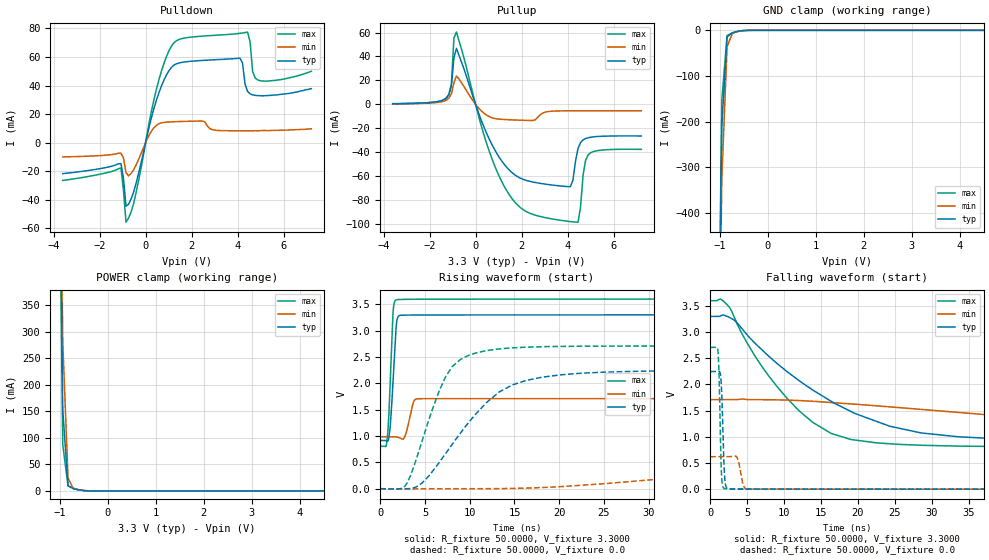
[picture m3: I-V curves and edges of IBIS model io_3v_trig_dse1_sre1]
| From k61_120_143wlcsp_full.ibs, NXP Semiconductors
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[Model]  io_3v_trig_dse1_sre1
|   Model io_3v_trig_dse1_sre1
| Library cells for typ/min/max conditions are connected as defined below:
|  pad - External Pad
|  ipp_do_3v - Core Input
|  ipp_obe_3v - Output Buffer Enable
|  esd_boost - vdd_s_3v
|  esd_trigger - vss_s_3v
|  ipp_ame_3v - vss_s_3v
|  ipp_dse_3v - vdd_s_3v
|  ipp_ina_3v - NC
|  ipp_ina_mux_3v - NC
|  ipp_ind_3v - NC
|  ipp_pue_3v - vss_s_3v
|  ipp_sre_3v - vdd_s_3v
|  tie_3v - vdd_s_3v
|  tie_hi - vdd_s_lv
|  vbuf_3v - vdd_s_3v
|  vdd_s_3v - vdd_s_3v
|  vdd_s_lv - vdd_s_lv
|  vss_bulk - vss_s_3v
|  vss_s_3v - vss_s_3v
| All other pins connected to ground
Model_type I/O
Polarity   Non-Inverting
Enable   Active-High
Vinl =   1.1550V
Vinh =   2.3100V
Vmeas =  1.6500V
Cref =   25.0000pF
Rref =   50.0000
Vref =   0.0V
C_comp   1.9033pF   1.7921pF   2.1182pF
[Temperature Range]   25.0000   0.1250k   -40.0000
[Voltage Range]   3.3000V   1.7100V   3.6000V
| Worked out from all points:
|   slope of the pulldown table from 0 to 0.495 V, typ, clamps not added: 16 ohm
|   slope of the pullup table from 0 to 0.495 V, typ, clamps not added: 19.9 ohm
|   GND clamp passes 1 mA (typ) near -0.54 V on its own axis
|   POWER clamp passes 1 mA (typ) near -0.53 V on its own axis
|   rising waveform, R_fixture 50.0000, V_fixture 3.3000: 20-80 % time 477ps typ, 573ps min, 395ps max; typ from 0.916 V to 3.3 V
|   rising waveform, R_fixture 50.0000, V_fixture 0.0: 20-80 % time 6.64ns typ, 30.7ns min, 3.47ns max; typ from 0 V to 2.25 V
|   falling waveform, R_fixture 50.0000, V_fixture 3.3000: 20-80 % time 14.8ns typ, 48ns min, 9.11ns max; typ from 3.3 V to 0.916 V
|   falling waveform, R_fixture 50.0000, V_fixture 0.0: 20-80 % time 304ps typ, 500ps min, 253ps max; typ from 2.25 V to 0 V
[Pulldown]
|Voltage   I(typ)   I(min)   I(max)
-3.6V     -21.69mA   -9.96mA    -26.46mA
-1.07V    -14.69mA   -7.404mA   -17.65mA
-850mV    -44.53mA   -20.93mA   -55.69mA
-520mV    -34.62mA   -18.99mA   -42.62mA
580mV     34.99mA    13.27mA    44.1mA
1.46V     55.81mA    14.78mA    72.31mA
4.1V      59.15mA    8.3mA      76.57mA
4.43V     35.88mA    8.3mA      77.43mA
4.54V     34.19mA    8.3mA      70.65mA
4.65V     33.46mA    8.3mA      49.92mA
4.87V     32.94mA    8.3mA      43.91mA
7.2V      37.8mA     9.7mA      50mA
[Pullup]
|Voltage   I(typ)   I(min)   I(max)
-3.6V     600uA      400uA      600uA
-1.27V    5.28mA     3.56mA     5.35mA
-1.05V    15.3mA     8.87mA     17.35mA
-940mV    39.22mA    18.09mA    55.5mA
-830mV    46.74mA    23.72mA    60.38mA
1.15V     -47.61mA   -12.48mA   -64.99mA
3.24V     -67.13mA   -5.816mA   -95.35mA
4.12V     -68.69mA   -5.32mA    -97.87mA
4.45V     -36.82mA   -5.29mA    -98.37mA
4.78V     -28.52mA   -5.28mA    -46.64mA
5V        -27.41mA   -5.28mA    -40.35mA
7.2V      -26.38mA   -5.36mA    -37.57mA
[GND_clamp]
|Voltage   I(typ)   I(min)   I(max)
-3.6V     -47.82A    -47.1A     -48.34A
-1.07V    -1.102A    -1.183A    -1.105A
-960mV    -210.7mA   -326mA     -154mA
-850mV    -14.47mA   -36.11mA   -11.11mA
-740mV    -5.262mA   -6.033mA   -5.843mA
-520mV    -636.9uA   -915.4uA   -467.5uA
-300mV    -2.578uA   -18.09uA   -370.9nA
7.2V      0A         0A         0A
[POWER_clamp]
|Voltage   I(typ)   I(min)   I(max)
-3.6V     36.98A     36.74A     37.19A
-1.05V    1.02A      1.161A     949.9mA
-940mV    152.3mA    280.6mA    87.35mA
-830mV    9.987mA    24.48mA    9.181mA
-720mV    4.227mA    4.408mA    5.116mA
-500mV    628.6uA    743.9uA    622.6uA
-390mV    66.57uA    164uA      29.9uA
7.2V      0A         0A         0A
[Ramp]
| variable   typ   min   max
dV/dt_r  1.3478/6.6433n   0.3719/30.7055n   1.6252/3.4740n
dV/dt_f  1.4301/14.8115n   0.4335/48.0367n   1.6764/9.1110n
R_load = 50.0000
[Rising Waveform]
R_fixture= 50.0000
V_fixture= 3.3000
V_fixture_min= 1.7100
V_fixture_max= 3.6000
|time   V(typ)   V(min)   V(max)
0s        916.5mV    987.2mV    806.1mV
650.6ps   913mV      987.2mV    805mV
931.5ps   941.1mV    987.7mV    1.321V
1.446ns   2.116V     987.7mV    3.391V
1.777ns   3.084V     983.2mV    3.584V
2.039ns   3.275V     972.7mV    3.592V
2.708ns   3.296V     974.6mV    3.594V
3.745ns   3.296V     1.659V     3.597V
4.46ns    3.297V     1.709V     3.598V
250ns     3.3V       1.71V      3.6V
[Rising Waveform]
R_fixture= 50.0000
V_fixture= 0.0
V_fixture_min= 0.0
V_fixture_max= 0.0
|time   V(typ)   V(min)   V(max)
0s        2.009nV    218.2nV    1.41nV
3.009ns   -219.1uV   -1.777mV   112mV
4.711ns   115.5mV    -189.2uV   928.5mV
6.575ns   496.1mV    -136.5uV   1.85V
8.035ns   842.2mV    -110.4uV   2.318V
11.88ns   1.637V     1.005mV    2.62V
14.36ns   1.934V     4.589mV    2.669V
25.16ns   2.214V     97.25mV    2.707V
76ns      2.246V     578mV      2.709V
250ns     2.246V     619.9mV    2.709V
[Falling Waveform]
R_fixture= 50.0000
V_fixture= 3.3000
V_fixture_min= 1.7100
V_fixture_max= 3.6000
|time   V(typ)   V(min)   V(max)
0s        3.3V       1.71V      3.6V
2.461ns   3.291V     1.71V      3.498V
7.044ns   2.656V     1.71V      2.333V
12.05ns   2.07V      1.693V     1.495V
16.36ns   1.681V     1.655V     1.065V
22.52ns   1.295V     1.593V     884.6mV
28.55ns   1.075V     1.524V     839mV
38.74ns   964.6mV    1.408V     814.7mV
86.94ns   917mV      1.075V     806mV
250ns     916.5mV    987.4mV    806.1mV
[Falling Waveform]
R_fixture= 50.0000
V_fixture= 0.0
V_fixture_min= 0.0
V_fixture_max= 0.0
|time   V(typ)   V(min)   V(max)
0s        2.246V     619.9mV    2.709V
1.039ns   2.248V     619.9mV    2.646V
1.215ns   2.248V     619.7mV    2.075V
1.383ns   2.193V     619.6mV    904.8mV
1.579ns   1.732V     619.5mV    152.8mV
1.894ns   356.7mV    619.3mV    10.97mV
2.096ns   61.58mV    619.3mV    5.077mV
3.634ns   1.8mV      605.6mV    1.153mV
5.311ns   835.3uV    1.1mV      672.1uV
250ns     -5.291nV   227.6nV    -4.024nV
